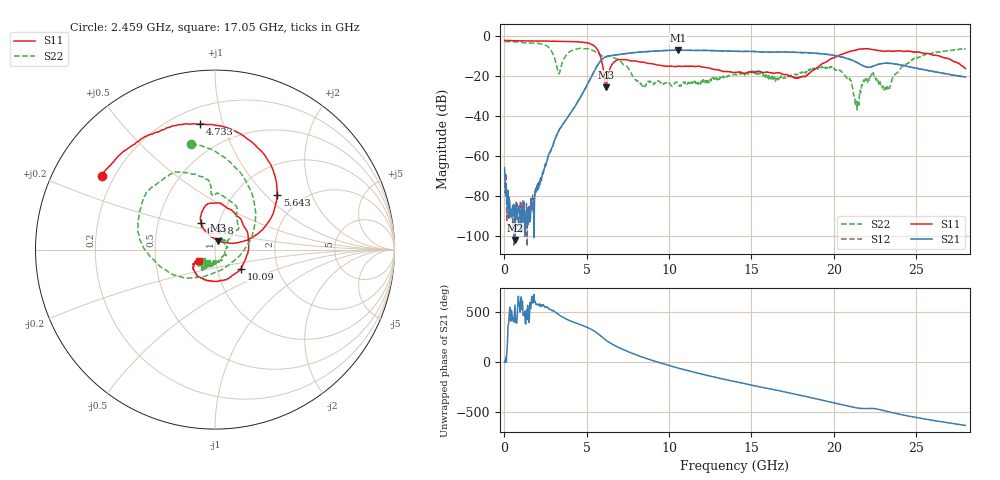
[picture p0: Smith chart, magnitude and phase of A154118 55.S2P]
!  2-Port S-parameters saved by WinCal
! VAR MeasName=S-Parameters (CALIBRATED_DATA) read from VNA (N5230A)
! VAR MeasDate=2015-9-10 14:39:22
! VAR NAME=A154118 55
! VAR FILENAME=A154118 55.S2P
! VAR DATE=2015-9-10 14:39:22
! VAR PHYS_PORTS=1,2
# Hz S DB R 50
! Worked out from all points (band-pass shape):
!   801 points, 10 MHz to 28 GHz, reference 50 ohm
!   highest |S21| = -7.02 dB at 10.54 GHz (marker M1); lowest = -101.7 dB at 639.8 MHz (marker M2)
!   |S21| within 3 dB of the highest: 6.282 GHz to 20.27 GHz (13.99 GHz wide, 105 % of centre)
!   lowest |S11| = -25.6 dB at 6.168 GHz (marker M3), VSWR 1.11, Z = 51.7 + j5.08 ohm
!   |S11| at or under -10 dB: 5.821 GHz to 20.22 GHz (14.39 GHz wide, 111 % of centre); 26.42 GHz to end of sweep
!   |S22| runs from -36.8 to -2.7 dB; largest |S21 - S12| = 0.0086
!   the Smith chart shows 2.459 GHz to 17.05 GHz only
!   S11 on the Smith chart (normalised r, x): 2.459 GHz: 0.15, +0.29; 4.733 GHz: 0.30, +0.84; 5.643 GHz: 1.51, +1.18; 6.448 GHz: 0.82, +0.25; 10.09 GHz: 1.30, -0.29; 17.05 GHz: 0.83, -0.11
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1e7  -2.15 179.7  -65.69 3.0  -68.85 61.0  -2.68 179.8
6.39775e8  -2.26 171.0  -101.75 -150.3  -84.79 90.7  -2.82 164.2
1.794362e9  -2.40 156.4  -100.49 -44.6  -82.18 -60.6  -3.45 135.2
2.459125e9  -2.47 146.9  -64.28 -168.2  -65.18 -168.7  -4.43 102.7
3.473762e9  -2.60 129.8  -44.93 94.4  -44.88 94.1  -14.31 -125.8
4.698325e9  -3.03 98.1  -29.35 8.5  -29.35 8.7  -6.09 136.5
4.733312e9  -3.06 96.6  -28.81 6.3  -28.83 6.3  -6.11 135.5
5.642988e9  -6.69 41.5  -14.69 -72.6  -14.64 -72.5  -8.33 95.1
6.1678e9  -25.59 69.0  -10.31 -142.3  -10.25 -142.4  -10.26 90.1
6.4477e9  -15.41 118.0  -9.78 -173.4  -9.72 -173.5  -10.20 84.2
7.777225e9  -12.40 72.1  -8.31 84.7  -8.28 84.4  -19.72 35.9
9.351662e9  -14.45 7.6  -7.37 -4.6  -7.32 -4.9  -22.53 46.3
1.00864e10  -14.94 -36.8  -7.09 -40.8  -7.05 -41.1  -24.23 5.7
1.054124e10  -14.95 -64.6  -7.02 -62.1  -6.98 -62.4  -23.63 -28.0
1.4005e10  -18.09 -147.9  -7.58 161.4  -7.56 160.9  -19.14 -118.3
1.704891e10  -19.14 -143.7  -7.90 57.0  -7.90 56.7  -21.04 -120.4
1.869332e10  -17.25 -95.1  -8.43 -1.7  -8.42 -2.2  -15.92 -114.4
2.04427e10  -9.21 -106.0  -10.33 -68.3  -10.31 -68.9  -17.61 -162.2
2.138736e10  -6.89 -125.9  -13.05 -101.9  -12.94 -102.9  -32.85 -155.1
2.233202e10  -6.67 -150.7  -15.23 -107.8  -15.18 -109.1  -18.78 -96.4
2.334666e10  -7.44 -160.0  -13.58 -141.5  -13.50 -142.9  -25.21 -35.3
2.8e10  -16.21 132.7  -20.39 81.5  -20.49 80.4  -6.07 -102.6
